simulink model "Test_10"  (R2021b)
settings: Solver=FixedStepAuto  StartTime=0.0  StopTime=60*60*6
undefined symbols (not defined in the file): Ion, Lithium
libraries: fl_lib x5, nesl_utility x5, ee_lib x2, spsBatteryLib x1, electricdrivelib x1, spsControlledVoltageSourceLib x1, spsDiodeLib x1, spspowerguiLib x1

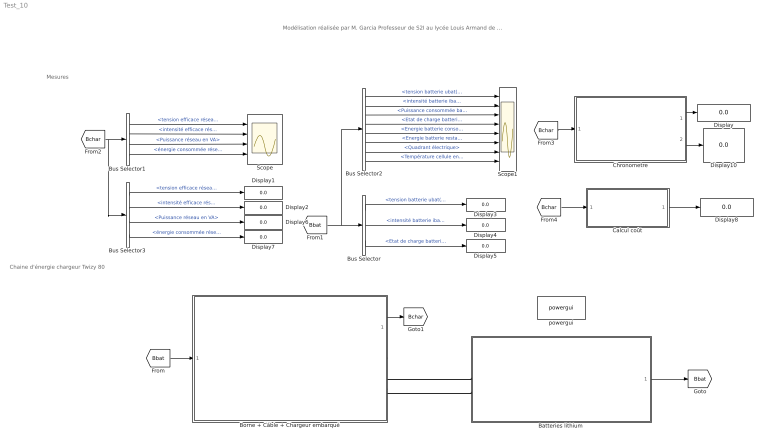
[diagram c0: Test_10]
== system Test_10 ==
  note: Mesures
  note: Chaine d'énergie chargeur Twizy 80
  note: Modélisation réalisée par M. Garcia Professeur de S2I au lycée Louis Armand de Nogent sur Marne
  Batteries lithium : Subsystem  mask{Ubat_n=54, Qbat_n=105, Soc_init=20, Soc_min=10, T_amb=0, T_init=35, Nb_cycles=1000, Nb_charge_mensuelle=20, Nb_mois=50}
      mask prompts: Ubat_n "Tension nominale batterie en V"; Qbat_n "Capacité nominale en A.h"; Soc_init "Etat de charge initial"; Soc_min "Seuil minimum en %"; T_amb "Température ambiante extérieure en °C"; T_init "Température initiale du bloc batteries en °C"; Nb_cycles "Durée de vie batterie en nombre de cycles"; Nb_charge_mensuelle "Nombre de recharges mensuelles"; Nb_mois "Nombre de mois d'utilisation"
  Borne + Câble + Chargeur embarqué : Subsystem  mask{Type_b=1, Vnom=230, P_borne=2.3, Se=2.5, Long=3, Pchargeur=1.8, rend_charg=85, Fp_charg=0.85, Ubat_n=54}
      mask prompts: Type_b "Type borne de charge (Monophasé :1 ; Triphasé : 3)"; Vnom "Tension nominale entre phase et neutre en Volt"; P_borne "Puissance borne de charge en kW"; Se "Section câble en mm²"; Long "Longueur câble en m"; Pchargeur "Puissance chargeur embarqué en kW"; rend_charg "Rendement du chargeur en %"; Fp_charg "Facteur de puissance du chargeur"; Ubat_n "Tension nominale batterie en V"
  Bus Selector : BusSelector  OutputSignals=tension batterie ubat(t),intensité batterie ibat(t),Etat de charge batterie soc(t) en %
  Bus Selector1 : BusSelector  OutputSignals=tension efficace réseau chargeur en V,intensité efficace réseau chargeur en A,Puissance réseau en VA,énergie consommée réseau en VAh
  Bus Selector2 : BusSelector  OutputSignals=tension batterie ubat(t),intensité batterie ibat(t),Puissance consommée batterie pbat(t) en W,Etat de charge batterie soc(t) en %,Energie batterie consommée wbat_cons(t) en Wh,Energie batterie restante wbat_rest(t) en Wh,Quadrant électrique,Température cellule en °C
  Bus Selector3 : BusSelector  OutputSignals=tension efficace réseau chargeur en V,intensité efficace réseau chargeur en A,Puissance réseau en VA,énergie consommée réseau en VAh
  Calcul coût : Subsystem  mask{P_Hc=0.1243}
      mask prompts: P_Hc "Coût du kWh en € TTC"
  Chronometre : Subsystem
  Display{,1..8,10} (10 alike) : Display
  Scope : Scope  NumInputPorts=4
  Scope1 : Scope  NumInputPorts=8
  powergui : spspowerguiLib/powergui  Priority=1  SimulationMode=Discrete  SampleTime=1  frequency=60  Iterations=50  frequencyindice=0  Pbase=100e6  ErrMax=1e-4  UnitsV=kV  UnitsW=MW  buscounter=0  FunctionMessages=off  echomessages=off  EnableUseOfTLC=off  CurrentSourceSwitches=off  DisableSnubberDevices=off  DisableRonSwitches=off  DisableVfSwitches=off  DisplayEquations=off  AutomaticDiscreteSolvers=off  SolverType=Tustin/Backward Euler (TBE)  Interpol=off  ExternalGateDelay=off  methode=off  Ts=100  x0status=blocks  SPID=on  SwTol=0  HookPort=off  NonlinearTolerance=1e-4  nMaxIteration=100  ContinueOnMaxIteration=off  RestoreLinks=warning  ResistiveCurrentMeasurement=off  Frange=[0:2:500]  Ylog=off  Xlog=on  ShowGrid=off  save=off  variable=ZData  structure=0  ZoomFFT=off  StartTime=0.0  cycles=1  DisplayStyle=1  fundamental=60  FreqAxis=off  MaxFrequency=1000  frequencyindicesteady=1  RmsSteady=1  display=off
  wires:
  Bus Selector/2 -> Display4/1  "<intensité batterie ibat(t)>"
  [Bbat] -> Bus Selector2/1, Bus Selector/1
  Bus Selector2/1 -> Scope1/1  "<tension batterie ubat(t)>"
  Bus Selector2/2 -> Scope1/2  "<intensité batterie ibat(t)>"
  Bus Selector2/3 -> Scope1/3  "<Puissance consommée batterie pbat(t) en W>"
  Bus Selector/1 -> Display3/1  "<tension batterie ubat(t)>"
  Bus Selector/3 -> Display5/1  "<Etat de charge batterie soc(t) en %>"
  Batteries lithium/1(Bus batterie) -> [Bbat]
  Bus Selector2/4 -> Scope1/4  "<Etat de charge batterie soc(t) en %>"
  Bus Selector2/7 -> Scope1/7  "<Quadrant électrique>"
  Bus Selector2/5 -> Scope1/5  "<Energie batterie consommée wbat_cons(t) en Wh>"
  Bus Selector2/6 -> Scope1/6  "<Energie batterie restante wbat_rest(t) en Wh>"
  [Bbat] -> Borne + Câble + Chargeur embarqué/1(bus_bat)
  Borne + Câble + Chargeur embarqué/1(Bus_chargeur) -> [Bchar]
  [Bchar] -> Bus Selector3/1, Bus Selector1/1
  Bus Selector1/1 -> Scope/1  "<tension efficace réseau chargeur en V>"
  Bus Selector1/2 -> Scope/2  "<intensité efficace réseau chargeur en A>"
  Bus Selector1/3 -> Scope/3  "<Puissance réseau en VA>"
  Bus Selector1/4 -> Scope/4  "<énergie consommée réseau en VAh>"
  Bus Selector3/1 -> Display1/1  "<tension efficace réseau chargeur en V>"
  Bus Selector3/2 -> Display2/1  "<intensité efficace réseau chargeur en A>"
  Bus Selector3/3 -> Display6/1  "<Puissance réseau en VA>"
  Bus Selector3/4 -> Display7/1  "<énergie consommée réseau en VAh>"
  Chronometre/1(Mesure temps de charge h) -> Display/1
  [Bchar] -> Chronometre/1(Bus chargeur)
  [Bchar] -> Calcul coût/1(Bus chargeur)
  Calcul coût/1(Cout en €) -> Display8/1
  Bus Selector2/8 -> Scope1/8  "<Température cellule en °C>"
  Chronometre/2(Mesure temps de charge HH mm ss) -> Display10/1
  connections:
  Borne + Câble + Chargeur embarqué/RConn2 -- Batteries lithium/LConn2
  Borne + Câble + Chargeur embarqué/RConn1 -- Batteries lithium/LConn1

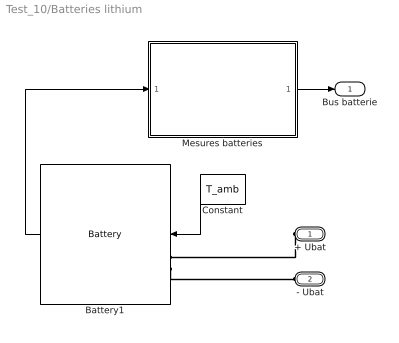
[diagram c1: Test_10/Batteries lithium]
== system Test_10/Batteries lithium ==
  Battery1 : spsBatteryLib/Battery  BatType=Lithium-Ion  ShowTempParam=on  ThermalPreset=no  ShowAgeParam=on  NomV=Ubat_n  NomQ=Qbat_n  SOC=Soc_init  Batt_Tr=30  PresetModel=on  MaxQ=105  MinV=40.5  FullV=62.8553  Dis_rate=45.6522  R=0.0051429  Normal_OP=94.9565  expZone="[58.3408       5.1587]"  current=[100 150 200]  Units=Time  Tci=T_init  NomT=25  T2=0  MaxQ2=Qbat_n/1.1517  FullV2=1.1933*Ubat_n  Normal_OP2=Ubat_n/1.1576  expZone2=[1.1338*Ubat_n Qbat_n/61]  Rca=0.06  ti=1000  Dp=0  Neq0=Nb_charge_mensuelle*Nb_mois  Tsim=30  Ta1=23  Qeol=0.9*Qbat_n  Reol=0.0126*1.2  Char_age=[0.38*Qbat_n, 0.495*Qbat_n]  Dis_age=[0.38*Qbat_n, 2*Qbat_n]  N1=Nb_cycles  N2=7*Nb_cycles  N3=Nb_cycles/1.5  N4=Nb_cycles*0.9733  Ta2=45  N5=Nb_cycles*0.655
  Constant : Constant  Value=T_amb
  Mesures batteries : Subsystem
  + Ubat : PMIOPort  Side=Left
  - Ubat : PMIOPort  Port=2  Side=Left
  Bus batterie : Outport  VectorParamsAs1DForOutWhenUnconnected=off
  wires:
  Battery1/1 -> Mesures batteries/1(Bus batteries)
  Mesures batteries/1(Bus_ batteries) -> Bus batterie/1
  Constant/1 -> Battery1/1
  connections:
  + Ubat/RConn1 -- Battery1/LConn1
  Battery1/LConn2 -- - Ubat/RConn1

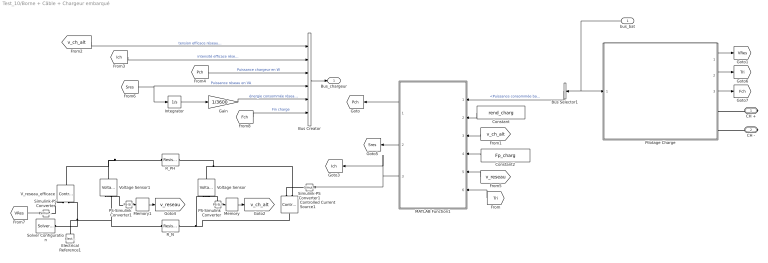
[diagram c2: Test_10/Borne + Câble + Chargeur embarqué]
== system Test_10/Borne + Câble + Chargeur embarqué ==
  bus_bat : Inport
  Bus Creator : BusCreator  Inputs=6
  Bus Selector1 : BusSelector  OutputSignals=Puissance consommée batterie pbat(t) en W
  Constant : Constant  Value=rend_charg
  Constant2 : Constant  Value=Fp_charg
  Controlled Current Source1 : fl_lib/Electrical/Electrical Sources/Controlled Current Source
  Electrical Reference1 : fl_lib/Electrical/Electrical Elements/Electrical Reference
  Gain : Gain  Gain=1/3600
  Integrator : Integrator
  MATLAB Function1 : MATLAB Function  TreatAsAtomicUnit=on
  Memory : Memory  InitialCondition=230
  Memory1 : Memory  InitialCondition=230
  PS-Simulink Converter : nesl_utility/PS-Simulink Converter  PhysicalDomain=network_engine_domain  SubClassName=ps_output  LeftPortType=input  RightPortType=output  PseudoPeriodic=off  Frequencies=[]  Unit=1  AffineConversion=off
  PS-Simulink Converter1 : nesl_utility/PS-Simulink Converter  PhysicalDomain=network_engine_domain  SubClassName=ps_output  LeftPortType=input  RightPortType=output  PseudoPeriodic=off  Frequencies=[]  Unit=1  AffineConversion=off
  Pilotage Charge : Subsystem
  R_N : ee_lib/Passive/Resistor  R=Long*22e-3/Se Ohm  R_tol=5  enable_R_tol=0  tol_distribution=1  nSigma=4  enable_operating_limits=0  operating_limit_action=2  max_working_voltage=100 V  power_rating=1 W  enable_faults=0  fault_action=1  R_faulted=inf Ohm  enable_temporal_fault=0  t_fault=1 s  enable_behavioral_fault=0  max_permissible_current=1 A  t_fail_on_current=1 s  noise_mode=0  sample_time=1e-3 s  repeatability=1  auto_seed=3499211588  user_seed=0  Tdevice=25 degC  power_derating_T1=70 degC  power_derating_T2=155 degC  operating_temperature_range_vec=[-50, 150] degC  alpha=3.93e-3 1/K  Tmeas=25 degC  thermal_mass=100 J/K  temperature_specify=off  temperature_priority=High  temperature=298.15 K  temperature_nominal_specify=off  temperature_nominal_unit=K  temperature_nominal_value=1
  R_PH : ee_lib/Passive/Resistor  R=Long*22e-3/Se Ohm  R_tol=5  enable_R_tol=0  tol_distribution=1  nSigma=4  enable_operating_limits=0  operating_limit_action=2  max_working_voltage=100 V  power_rating=1 W  enable_faults=0  fault_action=1  R_faulted=inf Ohm  enable_temporal_fault=0  t_fault=1 s  enable_behavioral_fault=0  max_permissible_current=1 A  t_fail_on_current=1 s  noise_mode=0  sample_time=1e-3 s  repeatability=1  auto_seed=3890346746  user_seed=0  Tdevice=25 degC  power_derating_T1=70 degC  power_derating_T2=155 degC  operating_temperature_range_vec=[-50, 150] degC  alpha=3.93e-3 1/K  Tmeas=25 degC  thermal_mass=100 J/K  temperature_specify=off  temperature_priority=High  temperature=298.15 K  temperature_nominal_specify=off  temperature_nominal_unit=K  temperature_nominal_value=1
  Simulink-PS Converter : nesl_utility/Simulink-PS Converter  PhysicalDomain=network_engine_domain  SubClassName=ps_input  LeftPortType=input  RightPortType=output  PseudoPeriodic=off  Frequencies=[]  NoiseDistribution=none  NoiseParameters=[]  Unit=V  AffineConversion=off  FilteringAndDerivatives=provide  SimscapeFilterOrder=1  InputFilterTimeConstant=0.001  UdotUserProvided=0
  Simulink-PS Converter1 : nesl_utility/Simulink-PS Converter  PhysicalDomain=network_engine_domain  SubClassName=ps_input  LeftPortType=input  RightPortType=output  PseudoPeriodic=off  Frequencies=[]  NoiseDistribution=none  NoiseParameters=[]  Unit=1  AffineConversion=off  FilteringAndDerivatives=provide  SimscapeFilterOrder=1  InputFilterTimeConstant=0.001  UdotUserProvided=0
  Solver Configuration : nesl_utility/Solver Configuration  PhysicalDomain=network_engine_domain  SubClassName=solver  LeftPortType=input  RightPortType=generic  Tones=[]  Harmonics=[]  SimulateNoise=off  Profile=off  UseLocalSampling=off  EnableSwitchedLinearOptims=on  FrequencyDomain=off  UseCCode=off  RelTol=0.001  AbsTol=1e-06  MinStep=1e-09  ToWorkspace=off  RevertToSquareIcSolve=off  NumHomotopyIterations=100  PhasorMode=off  PhasorModeNumHarmonics=1  DoDC=off  ResidualTolerance=1e-09  UseLocalSolver=off  LocalSolverChoice=NE_BACKWARD_EULER_ADVANCER  LocalSolverSampleTime=0.001  DoFixedCost=off  MaxNonlinIter=3  MaxModeIter=2  ComputeImpulses=off  ImpulseIterations=2  LinearAlgebra=auto  EquationFormulation=NE_TIME_EF  DelaysMemoryBudget=1024  AutomaticFiltering=on  FilteringTimeConstant=0.001  PartitionStorageMethod=AS_NEEDED  PartitionMemoryBudget=1024  PartitionMethod=ROBUST
  V_reseau_efficace : fl_lib/Electrical/Electrical Sources/Controlled Voltage Source
  Voltage Sensor : fl_lib/Electrical/Electrical Sensors/Voltage Sensor
  Voltage Sensor1 : fl_lib/Electrical/Electrical Sensors/Voltage Sensor
  CH + : PMIOPort  Side=Right
  CH - : PMIOPort  Port=2  Side=Right
  Bus_chargeur : Outport  VectorParamsAs1DForOutWhenUnconnected=off
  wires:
  Constant/1 -> MATLAB Function1/2(rend_chargeur)
  bus_bat/1 -> Bus Selector1/1, Pilotage Charge/1(Bus Bat)
  Bus Selector1/1 -> MATLAB Function1/1(P_bat)  "<Puissance consommée batterie pbat(t) en W>"
  [v_ch_alt] -> MATLAB Function1/3(Vch)
  PS-Simulink Converter/1 -> Memory/1
  Memory/1 -> [v_ch_alt]
  MATLAB Function1/1(Pch) -> [Pch]
  [v_ch_alt] -> Bus Creator/1  "tension efficace réseau chargeur en V"
  [Ich] -> Bus Creator/2  "intensité efficace réseau chargeur en A"
  [Pch] -> Bus Creator/3  "Puissance chargeur en W"
  Gain/1 -> Bus Creator/5  "énergie consommée réseau en VAh"
  Bus Creator/1 -> Bus_chargeur/1
  Constant2/1 -> MATLAB Function1/4(Fp_ch)
  Integrator/1 -> Gain/1
  Memory1/1 -> [v_reseau]
  PS-Simulink Converter1/1 -> Memory1/1
  [v_reseau] -> MATLAB Function1/5(V_reseau)
  MATLAB Function1/2(Sreseau) -> [Sres]
  [Sres] -> Integrator/1, Bus Creator/4  "Puissance réseau en VA"
  MATLAB Function1/3(I_alt_ch) -> Simulink-PS Converter1/1, [Ich]
  Pilotage Charge/1(Vreseau) -> [VRes]
  [VRes] -> Simulink-PS Converter/1
  Pilotage Charge/2(Triphase) -> [Tri]
  [Tri] -> MATLAB Function1/6(Tri)
  Pilotage Charge/3(Fin_charge) -> [Fch]
  [Fch] -> Bus Creator/6  "Fin charge"
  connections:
  R_PH/LConn1 -- V_reseau_efficace/LConn1 -- Voltage Sensor1/LConn1
  R_N/RConn1 -- Controlled Current Source1/LConn1 -- Voltage Sensor/RConn2
  Controlled Current Source1/RConn1 -- Simulink-PS Converter1/RConn1
  PS-Simulink Converter/LConn1 -- Voltage Sensor/RConn1
  Controlled Current Source1/RConn2 -- Voltage Sensor/LConn1 -- R_PH/RConn1
  PS-Simulink Converter1/LConn1 -- Voltage Sensor1/RConn1
  Pilotage Charge/RConn2 -- CH -/RConn1
  Voltage Sensor1/RConn2 -- V_reseau_efficace/RConn2 -- Solver Configuration/RConn1 -- Electrical Reference1/LConn1 -- R_N/LConn1
  Simulink-PS Converter/RConn1 -- V_reseau_efficace/RConn1
  Pilotage Charge/RConn1 -- CH +/RConn1

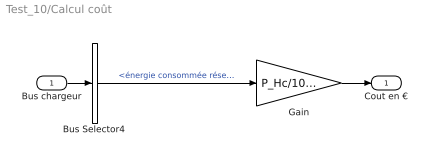
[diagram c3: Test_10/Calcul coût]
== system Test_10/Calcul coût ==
  Bus chargeur : Inport
  Bus Selector4 : BusSelector  OutputSignals=énergie consommée réseau en VAh
  Gain : Gain  Gain=P_Hc/1000
  Cout en € : Outport  VectorParamsAs1DForOutWhenUnconnected=off
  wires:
  Bus Selector4/1 -> Gain/1  "<énergie consommée réseau en VAh>"
  Gain/1 -> Cout en €/1
  Bus chargeur/1 -> Bus Selector4/1

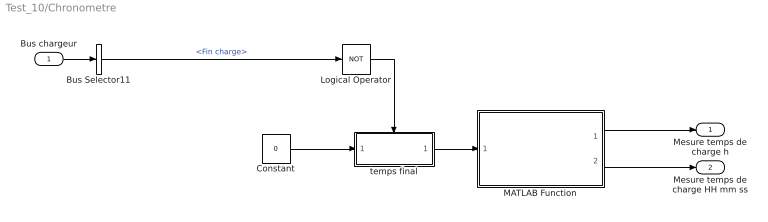
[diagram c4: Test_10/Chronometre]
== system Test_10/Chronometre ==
  Bus chargeur : Inport
  Bus Selector11 : BusSelector  OutputSignals=Fin charge
  Constant : Constant  Value=0
  Logical Operator : Logic  Operator=NOT  AllPortsSameDT=off  OutDataTypeStr=boolean
  MATLAB Function : MATLAB Function  TreatAsAtomicUnit=on
  temps final : Subsystem
  Mesure temps de charge h : Outport  VectorParamsAs1DForOutWhenUnconnected=off
  Mesure temps de charge HH mm ss : Outport  Port=2  VectorParamsAs1DForOutWhenUnconnected=off
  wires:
  Bus Selector11/1 -> Logical Operator/1  "<Fin charge>"
  Bus chargeur/1 -> Bus Selector11/1
  Constant/1 -> temps final/1(tps_init)
  temps final/1(delta_tps) -> MATLAB Function/1(u)
  MATLAB Function/2(HH_M_SS) -> Mesure temps de charge HH mm ss/1
  MATLAB Function/1(dec) -> Mesure temps de charge h/1
  Logical Operator/1 -> temps final/Enable

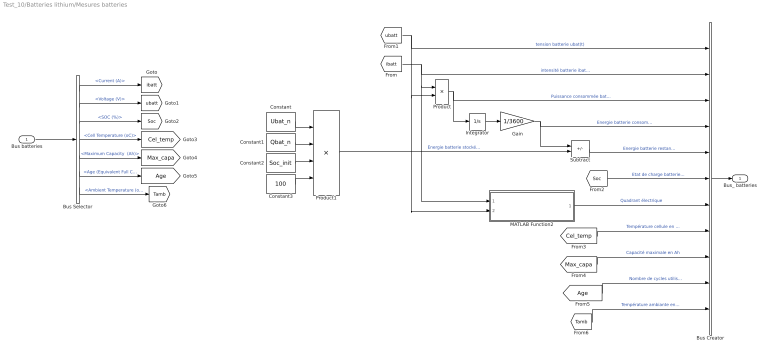
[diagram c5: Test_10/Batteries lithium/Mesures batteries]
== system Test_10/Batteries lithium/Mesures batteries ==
  Bus batteries : Inport
  Bus Creator : BusCreator  Inputs=11
  Bus Selector : BusSelector  OutputSignals="Current (A),Voltage (V),SOC (%),Cell Temperature (oC),Maximum Capacity  (Ah),Age (Equivalent Full Cycles),Ambient Temperature (oC)"
  Constant : Constant  Value=Ubat_n
  Constant1 : Constant  Value=Qbat_n
  Constant2 : Constant  Value=Soc_init
  Constant3 : Constant  Value=100
  Gain : Gain  Gain=1/3600
  Integrator : Integrator
  MATLAB Function2 : MATLAB Function  TreatAsAtomicUnit=on
  Product : Product
  Product1 : Product  Inputs=***/
  Subtract : Sum  Inputs=-+
  Bus_ batteries : Outport  VectorParamsAs1DForOutWhenUnconnected=off
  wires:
  Bus batteries/1 -> Bus Selector/1
  Product/1 -> Bus Creator/3, Integrator/1  "Puissance consommée batterie pbat(t) en W"
  Bus Creator/1 -> Bus_ batteries/1
  Integrator/1 -> Gain/1
  Gain/1 -> Bus Creator/4, Subtract/1  "Energie batterie consommée wbat_cons(t) en Wh"
  [ibatt] -> Bus Creator/2, MATLAB Function2/1(I_bat), Product/1  "intensité batterie ibat(t)"
  Bus Selector/1 -> [ibatt]  "<Current (A)>"
  Bus Selector/2 -> [ubatt]  "<Voltage (V)>"
  [ubatt] -> MATLAB Function2/2(U_bat), Product/2, Bus Creator/1  "tension batterie ubat(t)"
  Bus Selector/3 -> [Soc]  "<SOC (%)>"
  [Soc] -> Bus Creator/6  "Etat de charge batterie soc(t) en %"
  MATLAB Function2/1(Quadrant_elec) -> Bus Creator/7  "Quadrant électrique"
  Constant/1 -> Product1/1
  Constant1/1 -> Product1/2
  Constant2/1 -> Product1/3
  Constant3/1 -> Product1/4
  Subtract/1 -> Bus Creator/5  "Energie batterie restante wbat_rest(t) en Wh"
  Product1/1 -> Subtract/2  "Energie batterie stockée wstock_batt(t) en Wh"
  Bus Selector/4 -> [Cel_temp]  "<Cell Temperature (oC)>"
  Bus Selector/5 -> [Max_capa]  "<Maximum Capacity  (Ah)>"
  Bus Selector/6 -> [Age]  "<Age (Equivalent Full Cycles)>"
  [Cel_temp] -> Bus Creator/8  "Température cellule en °C"
  [Max_capa] -> Bus Creator/9  "Capacité maximale en Ah"
  [Age] -> Bus Creator/10  "Nombre de cycles utilisés"
  Bus Selector/7 -> [Tamb]  "<Ambient Temperature (oC)>"
  [Tamb] -> Bus Creator/11  "Température ambiante en °C"

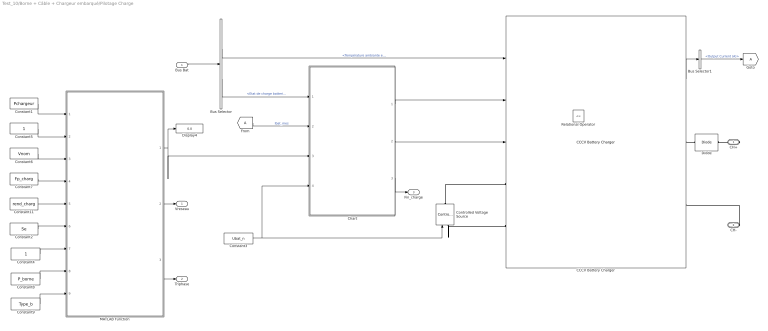
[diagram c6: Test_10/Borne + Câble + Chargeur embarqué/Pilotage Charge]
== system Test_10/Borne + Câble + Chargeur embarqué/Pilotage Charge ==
  Bus Bat : Inport
  Bus Selector : BusSelector  OutputSignals=Température ambiante en °C,Etat de charge batterie soc(t) en %
  Bus Selector1 : BusSelector  OutputSignals=Output Current (A)
  CCCV Battery Charger : electricdrivelib/Extra Sources/CCCV Battery Charger  Preset=Custom specifications  P_nom=Pchargeur  s_type=DC  n_connect=off  eff_volt=63  in_freq=60  in_I_ripple=10  in_I_freq=1000  EFF_en=on  EFF_val=[0.627 0.803 0.855 0.871 0.872 0.864]  EFF_fu=[0.063 0.177 0.293 0.483 0.674 0.914]  THD_en=on  I_THD_val=[0.327 0.394 0.394 0.351 0.289 0.265]  I_THD_fu=[0.056 0.136 0.194 0.303 0.555 0.916]  H_DIST_rt=[0.199 1.297 0.328 0.029 0.416 0.200]  H_DIST_fr=[3 5 7 9 11 13]  PF_en=on  PF_val=[0.316 0.532 0.662 0.731 0.780 0.792]  PF_fu=[0.067 0.230 0.445 0.625 0.794 0.919]  Out_mode=Constant Current - Constant Voltage (CCCV)  DynInT=on  I_cst=10  V_cst=138  ABS_en=off  V_abs=142  ABS_end=Time based  ABS_time=3600  ABS_i=40  ripple=0.05  swF=1  overshoot=0  stable_t=5  VoltComp=on  V_comp=-0.18  nom_temp=20
  Chart : Stateflow chart  TreatAsAtomicUnit=on
  Constant1 : Constant  Value=Pchargeur
  Constant11 : Constant  Value=rend_charg
  Constant2 : Constant  Value=Se
  Constant3 : Constant  Value=Ubat_n
  Constant4 : Constant
  Constant5 : Constant
  Constant6 : Constant  Value=Vnom
  Constant7 : Constant  Value=Fp_charg
  Constant8 : Constant  Value=P_borne
  Constant9 : Constant  Value=Type_b
  Controlled Voltage Source : spsControlledVoltageSourceLib/Controlled Voltage Source  Initialize=on  Source_Type=DC  Amplitude=Ubat_n  Phase=0  Frequency=0  Measurements=None
  Diode : spsDiodeLib/Diode  Ron=0.001  Lon=0  Vf=0.8  IC=0  UseSnubber=0  Rs=500  Cs=250e-9  Measurements=off
  Display4 : Display
  From : From
  Goto : Goto
  MATLAB Function : MATLAB Function  TreatAsAtomicUnit=on
  Relational Operator : RelationalOperator  Operator=<=  OutDataTypeStr=boolean  RndMeth=Simplest
  CH+ : PMIOPort  Side=Right
  CH- : PMIOPort  Port=2  Side=Right
  Vreseau : Outport
  Triphase : Outport  Port=2
  Fin_charge : Outport  Port=3
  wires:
  CCCV Battery Charger/1 -> Bus Selector1/1
  Constant11/1 -> MATLAB Function/5(rend_charg)
  Constant2/1 -> MATLAB Function/6(Se)
  Constant9/1 -> MATLAB Function/9(Type_b)
  Constant4/1 -> MATLAB Function/7(Nb_fil)
  Constant6/1 -> MATLAB Function/3(Vnom)
  Constant8/1 -> MATLAB Function/8(P_borne)
  Constant5/1 -> MATLAB Function/2(Type_c)
  Constant1/1 -> MATLAB Function/1(Pchargeur)
  Constant7/1 -> MATLAB Function/4(Fp_charg)
  Chart/1(Icch) -> CCCV Battery Charger/2
  MATLAB Function/1(Pmax_auto) -> Chart/3(Pmax_auto), Display4/1
  Bus Bat/1 -> Bus Selector/1
  Bus Selector/1 -> CCCV Battery Charger/1  "<Température ambiante en °C>"
  MATLAB Function/2(V) -> Vreseau/1
  MATLAB Function/3(Triphase) -> Triphase/1
  Bus Selector1/1 -> Goto/1  "<Output Current (A)>"
  From/1 -> Chart/2(Ibat_mes)  "Ibat_mes"
  Bus Selector/2 -> Chart/1(Soc)  "<Etat de charge batterie soc(t) en %>"
  Constant3/1 -> Chart/4(Ubat_n), Controlled Voltage Source/1
  Chart/3(Fin_charge) -> Fin_charge/1
  Chart/2(Uccv) -> CCCV Battery Charger/3
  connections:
  CCCV Battery Charger/RConn1 -- Diode/LConn1
  CH-/RConn1 -- CCCV Battery Charger/RConn2
  Controlled Voltage Source/LConn1 -- CCCV Battery Charger/LConn2
  Controlled Voltage Source/RConn1 -- CCCV Battery Charger/LConn1
  Diode/RConn1 -- CH+/RConn1

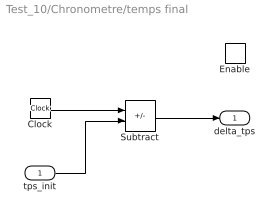
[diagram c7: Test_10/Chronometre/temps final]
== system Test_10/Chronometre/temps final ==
  tps_init : Inport
  Enable : EnablePort
  Clock : Clock
  Subtract : Sum  Inputs=+-
  delta_tps : Outport  VectorParamsAs1DForOutWhenUnconnected=off
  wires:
  Clock/1 -> Subtract/1
  tps_init/1 -> Subtract/2
  Subtract/1 -> delta_tps/1

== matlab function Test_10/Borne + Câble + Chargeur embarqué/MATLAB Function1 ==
function [Pch,Sreseau,I_alt_ch]= fcn(P_bat,rend_chargeur,Vch,Fp_ch, V_reseau, Tri)
Pch = -P_bat/(rend_chargeur/100);
if Tri==1
    I_alt_ch = Pch/(3*Vch*Fp_ch);
    Sreseau = I_alt_ch*V_reseau*3;
else
    I_alt_ch = Pch/(Vch*Fp_ch);
    Sreseau = I_alt_ch*V_reseau;
end
end

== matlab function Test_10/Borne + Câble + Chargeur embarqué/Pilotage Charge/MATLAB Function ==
function [Pmax_auto,V,Triphase] = fcndata(Pchargeur, Type_c, Vnom, Fp_charg, rend_charg, Se, Nb_fil, P_borne, Type_b)

switch Pchargeur
    case 1
        P_chargeur=1800;
    case 2
        P_chargeur=2300;
    case 3
        P_chargeur=3700;
    case 4
        P_chargeur=7400;
    case 5
        P_chargeur=11000;        
    otherwise
        P_chargeur=22000;
end

switch P_borne
    case 1
        Pborne=2300;
    case 2
        Pborne=3700;
    case 3
        Pborne=7400;
    case 4
        Pborne=11000;
    otherwise
        Pborne=22000;
end
switch Se
    case 1
        I_cable=13;
    case 2
        I_cable=20;
    case 3
        I_cable=32;
    otherwise
        I_cable=63;
end
switch Vnom
    case 1
        V=230;
    case 2
        V=240;
    otherwise
        V=250;
end

if Type_c==1
    I_chargeur=P_chargeur/(V*Fp_charg);
else
    I_chargeur=P_chargeur/(3*V*Fp_charg);
end
if Type_b==1
    I_borne=Pborne/(V*Fp_charg);
else
    I_borne=Pborne/(3*V*Fp_charg);
end

if I_chargeur<=I_cable
    if I_chargeur<=I_borne
        I_lim=I_chargeur;
    else
        I_lim=I_borne;
    end
else
    if I_cable<=I_borne
        I_lim=I_cable;
    else
        I_lim=I_borne;
    end
end

if Nb_fil==2&&Type_b==2&&Type_c==2
    Pmax_auto = 3*V*I_lim*Fp_charg*rend_charg/100;
    Triphase=1;
else
    Pmax_auto = V*I_lim*Fp_charg*rend_charg/100;
    Triphase=0;
end

end

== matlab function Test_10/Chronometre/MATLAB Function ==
function [dec,HH_M_SS]= fcn(u)
dec=u/3600;
hour = floor(dec);
min=floor((dec-hour)*60);
sec=floor(rem((dec-hour)*60,1)*60);
HH_M_SS=[hour,min,sec];
end

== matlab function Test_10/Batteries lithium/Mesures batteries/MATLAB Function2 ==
function Quadrant_elec = fcn(I_bat,U_bat)
if U_bat > 0.8
    if I_bat > 0.3
        Quadrant_elec = 1;
    elseif I_bat < -0.5
        Quadrant_elec = 4;
    else
        Quadrant_elec = 0;
    end
elseif U_bat < -0.8
    if I_bat > 0.5
        Quadrant_elec = 2;
    elseif I_bat < -0.5
        Quadrant_elec = 3;
    else
        Quadrant_elec = 0;
    end
else
    Quadrant_elec = 0;
end
end

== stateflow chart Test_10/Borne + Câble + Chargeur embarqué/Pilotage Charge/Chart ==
  state CH0
    entry:
    Icch=Pmax_auto/Ubat_n;
    Uccv=Ubat_n*1.25;
  state CH01
    entry:
    Uccv=Ubat_n*1.15;
  state CH02
    Icch=0;
    Fin_charge=1;
  (default) -> CH0 : {Fin_charge=0;}
  CH0 -> CH01 : [Soc==100]
  CH01 -> CH02 : [Ibat_mes<=0.05*Icch]
  data: Icch output; Soc input; Uccv output; Ibat_mes input; Pmax_auto input; Ubat_n input; Fin_charge output
